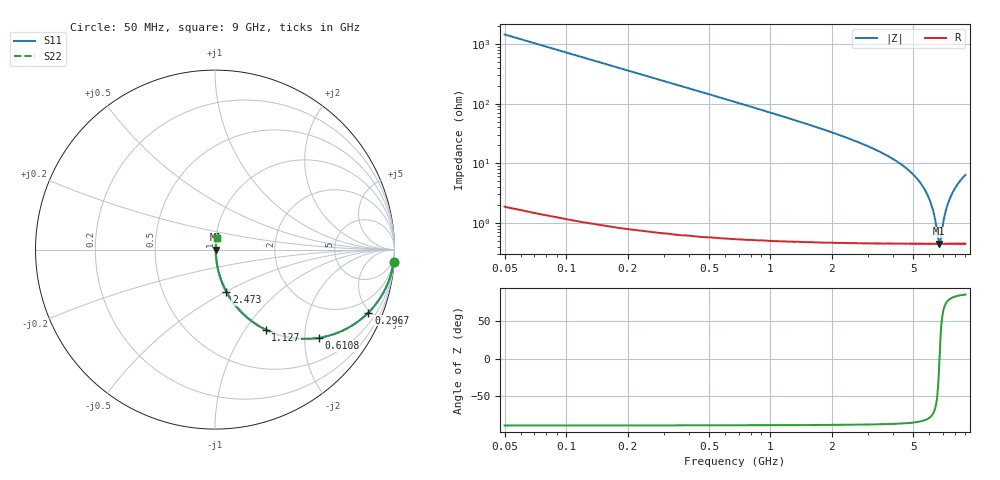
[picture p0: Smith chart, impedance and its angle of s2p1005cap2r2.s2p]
!	AVX	Thin	Film	Operation
!	Date:	March 2012
!	Description: Ultra-Miniature 01005 Size ACCU - P® Thin Film RF / Microwave Capacitor
!	Part Number:  C005YK2R2ABSTR
!	Serial	Measurements
#	MHz	S	db	R	50
!	S11	S21	S12	S22
!	dB	Phase	dB	Phase	dB	Phase	dB	Phase
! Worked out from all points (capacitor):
!   400 points, 50 MHz to 9 GHz, reference 50 ohm
!   read as one part in series: C = 2.2 pF near 94.86 MHz
!   lowest |Z| = 449 mohm at 6.712 GHz (marker M1)
!   series resonance near 6.72 GHz, so ESL is about 250 pH
!   S11 on the Smith chart (normalised r, x): 50 MHz: 1, -29; 296.7 MHz: 1.01, -4.87; 610.8 MHz: 1.01, -2.35; 1.127 GHz: 1.01, -1.25; 2.473 GHz: 1.01, -0.51; 9 GHz: 1.01, +0.13
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50  -0.02 -4.0  -23.23 86.0  -23.23 86.0  -0.02 -4.0
94.862  -0.08 -7.5  -17.72 82.4  -17.72 82.4  -0.08 -7.5
139.724  -0.16 -10.9  -14.44 79.0  -14.44 79.0  -0.16 -10.9
207.018  -0.35 -16.0  -11.21 73.9  -11.21 73.9  -0.35 -16.0
296.742  -0.69 -22.3  -8.41 67.5  -8.41 67.5  -0.69 -22.3
431.328  -1.34 -30.9  -5.80 58.9  -5.80 58.9  -1.34 -30.9
610.777  -2.39 -40.3  -3.79 49.4  -3.79 49.4  -2.39 -40.3
1126.692  -5.55 -57.7  -1.46 31.8  -1.46 31.8  -5.55 -57.7
1552.882  -7.92 -65.7  -0.81 23.7  -0.81 23.7  -7.92 -65.7
2472.556  -12.24 -74.8  -0.31 14.1  -0.31 14.1  -12.24 -74.8
3055.764  -14.71 -78.0  -0.19 10.6  -0.19 10.6  -14.71 -78.0
4536.216  -21.29 -82.1  -0.07 4.9  -0.07 4.9  -21.29 -82.1
5411.028  -26.57 -81.9  -0.05 2.7  -0.05 2.7  -26.57 -81.9
6016.667  -32.35 -78.0  -0.04 1.4  -0.04 1.4  -32.35 -78.0
6353.133  -37.84 -69.0  -0.04 0.7  -0.04 0.7  -37.84 -69.0
6644.737  -45.93 -28.2  -0.04 0.1  -0.04 0.1  -45.93 -28.2
6712.03  -47.03 -3.1  -0.04 0.0  -0.04 0.0  -47.03 -3.1
6779.323  -46.31 23.0  -0.04 -0.1  -0.04 -0.1  -46.31 23.0
7138.221  -37.26 70.3  -0.04 -0.7  -0.04 -0.7  -37.26 70.3
7519.549  -32.19 78.2  -0.04 -1.4  -0.04 -1.4  -32.19 78.2
8125.188  -27.71 81.5  -0.05 -2.3  -0.05 -2.3  -27.71 81.5
9000  -23.94 82.4  -0.06 -3.6  -0.06 -3.6  -23.94 82.4
